| Teraspeed Modeling Services.
| http://www.teraspeed.com
[IBIS Ver]   3.2
[Comment Char] |_char
[File Name]   lpc1788fbd208.ibs
[File Rev]   3.0
[Source]  Measured and created by Teraspeed Consulting Group LLC
[Date]   04-01-2011
[Notes]   Quality Check of this IBIS model: Model Passes IBIS Check
   Model parses into ICX IS. Simulation done with Hyperlynx.
   1. MIN TYP MAX information is based on Temperature and Voltage
   characteristics only.
   2. Package data measured using Tektronix IConnect Software.
[Disclaimer]
| NXP Semiconductors warrants and represents that the IBIS models
| identified herein are owned by NXP Semiconductors (NXP).  The
| models provided are not warranted as fully representing all of the
| operating characteristics and specifications of the semiconductor
| products to which the models relate.  Moreover, unless there is a
| signed, written agreement to the contrary, these models are furnished
| on an "as is" basis without support or warranty of any kind, either
| expressed or implied, regarding the use thereof, and NXP
| specifically disclaims all implied warranties of merchantability and
| fitness of the models for any purpose.
| NXP does not assume any liability arising out of the application
| or use of these IBIS models including infringement of patents and
| copyrights, nor does NXP convey any license under its patents and
| copyrights or the rights of others.
| NXP provides IBIS models as a service to our customers.  You and
| your company shall not distribute, convey, sell, or give these models
| to anyone else without receiving prior written permission from
| NXP.
[Copyright]  NXP Semiconductors 2011. All rights reserved.
|   LPC177x_8x (208 LQFP package) IBIS Model
|   IBIS Model Created by Teraspeed Consulting Group
|   www.teraspeed.com
[Component] LPC1788FBD208
[Manufacturer] NXP Semiconductors
[Package]
| variable   typ   min   max
| lqfp208
R_pkg  1.000E-02  1.000E-02  1.000E-02
L_pkg  8.067E-09  6.742E-09  9.392E-09
C_pkg  1.248E-12  1.080E-12  1.417E-12
[Pin] signal_name  model_name  R_pin  L_pin C_pin
1   P3_12   io_pad   1.000E-02  9.392E-09  1.417E-12
2   JTAG_TDO   tri_pad   1.000E-02  9.286E-09  1.404E-12
3   P3_3   io_pad   1.000E-02  9.180E-09  1.390E-12
4   JTAG_TDI   in_pu   1.000E-02  9.074E-09  1.377E-12
5   P3_28   io_pad   1.000E-02  8.968E-09  1.363E-12
6   JTAG_TMS   in_pu   1.000E-02  8.862E-09  1.350E-12
7   P3_13   io_pad   1.000E-02  8.756E-09  1.336E-12
8   JTAG_*TRST   in_pu   1.000E-02  8.650E-09  1.323E-12
9   P5_0   io_pad   1.000E-02  8.544E-09  1.309E-12
10   JTAG_TCK   in_tck   1.000E-02  8.438E-09  1.296E-12
11   P3_29   io_pad   1.000E-02  8.332E-09  1.282E-12
12   P0_26   io_pad   1.000E-02  8.226E-09  1.269E-12
13   P3_4   io_pad   1.000E-02  8.120E-09  1.255E-12
14   P0_25   io_pad   1.000E-02  8.014E-09  1.242E-12
15   Vdd(3v3)   POWER   1.000E-02  7.908E-09  1.228E-12
16   P0_24   io_pad   1.000E-02  7.802E-09  1.215E-12
17   P3_5   io_pad   1.000E-02  7.696E-09  1.201E-12
18   P0_23   io_pad   1.000E-02  7.590E-09  1.188E-12
19   P3_30   io_pad   1.000E-02  7.484E-09  1.174E-12
20   Vdda   POWER   1.000E-02  7.378E-09  1.161E-12
21   P3_14   io_pad   1.000E-02  7.272E-09  1.147E-12
22   Vssa   GND   1.000E-02  7.166E-09  1.134E-12
23   P3_6   io_pad   1.000E-02  7.060E-09  1.120E-12
24   VREFP   term   1.000E-02  6.954E-09  1.107E-12
25   P3_31   io_pad   1.000E-02  6.848E-09  1.093E-12
26   Vdd(reg)(3v3)   POWER   1.000E-02  6.742E-09  1.080E-12
27   P3_7   io_pad   1.000E-02  6.742E-09  1.080E-12
28   P3_15   io_pad   1.000E-02  6.848E-09  1.093E-12
29   *RSTOUT   out_pad   1.000E-02  6.954E-09  1.107E-12
30   P5_1   io_pad   1.000E-02  7.060E-09  1.120E-12
31   P2_30   io_pad   1.000E-02  7.166E-09  1.134E-12
32   Vss(reg)   GND   1.000E-02  7.272E-09  1.147E-12
33   VSS   GND   1.000E-02  7.378E-09  1.161E-12
34   RTCX1   term   1.000E-02  7.484E-09  1.174E-12
35   *RESET   in_resetb   1.000E-02  7.590E-09  1.188E-12
36   RTCX2   term   1.000E-02  7.696E-09  1.201E-12
37   RTC_ALARM   rtc_alarm   1.000E-02  7.802E-09  1.215E-12
38   Vbat   POWER   1.000E-02  7.908E-09  1.228E-12
39   P2_31   io_pad   1.000E-02  8.014E-09  1.242E-12
40   P1_31   io_pad   1.000E-02  8.120E-09  1.255E-12
41   P0_12   io_pad   1.000E-02  8.226E-09  1.269E-12
42   P1_30   io_pad   1.000E-02  8.332E-09  1.282E-12
43   P2_29   io_pad   1.000E-02  8.438E-09  1.296E-12
44   XTAL1   term   1.000E-02  8.544E-09  1.309E-12
45   P0_13   io_pad   1.000E-02  8.650E-09  1.323E-12
46   XTAL2   term   1.000E-02  8.756E-09  1.336E-12
47   P2_27   io_pad   1.000E-02  8.862E-09  1.350E-12
48   P0_28   od2_pad   1.000E-02  8.968E-09  1.363E-12
49   P2_28   io_pad   1.000E-02  9.074E-09  1.377E-12
50   P0_27   od2_pad   1.000E-02  9.180E-09  1.390E-12
51   P0_31   io_pad   1.000E-02  9.286E-09  1.404E-12
52   USB_D2N   io_pad   1.000E-02  9.392E-09  1.417E-12
53   P2_24   io_pad   1.000E-02  9.392E-09  1.417E-12
54   P2_25   io_pad   1.000E-02  9.286E-09  1.404E-12
55   P3_26   io_pad   1.000E-02  9.180E-09  1.390E-12
56   P3_25   io_pad   1.000E-02  9.074E-09  1.377E-12
57   P2_26   io_pad   1.000E-02  8.968E-09  1.363E-12
58   P3_24   io_pad   1.000E-02  8.862E-09  1.350E-12
59   P2_18   io_pad   1.000E-02  8.756E-09  1.336E-12
60   Vdd(3v3)   POWER   1.000E-02  8.650E-09  1.323E-12
61   P0_29   io_pad   1.000E-02  8.544E-09  1.309E-12
62   P0_30   io_pad   1.000E-02  8.438E-09  1.296E-12
63   VSS   GND   1.000E-02  8.332E-09  1.282E-12
64   P2_23   io_pad   1.000E-02  8.226E-09  1.269E-12
65   P3_23   io_pad   1.000E-02  8.120E-09  1.255E-12
66   P1_18   io_pad   1.000E-02  8.014E-09  1.242E-12
67   P2_19   io_pad   1.000E-02  7.908E-09  1.228E-12
68   P1_19   io_pad   1.000E-02  7.802E-09  1.215E-12
69   P0_14   io_pad   1.000E-02  7.696E-09  1.201E-12
70   P1_20   io_pad   1.000E-02  7.590E-09  1.188E-12
71   Vdd(3v3)   POWER   1.000E-02  7.484E-09  1.174E-12
72   P1_21   io_pad   1.000E-02  7.378E-09  1.161E-12
73   P2_20   io_pad   1.000E-02  7.272E-09  1.147E-12
74   P1_22   io_pad   1.000E-02  7.166E-09  1.134E-12
75   P4_0   io_pad   1.000E-02  7.060E-09  1.120E-12
76   P1_23   io_pad   1.000E-02  6.954E-09  1.107E-12
77   VSS   GND   1.000E-02  6.848E-09  1.093E-12
78   P1_24   io_pad   1.000E-02  6.742E-09  1.080E-12
79   P4_1   io_pad   1.000E-02  6.742E-09  1.080E-12
80   P1_25   io_pad   1.000E-02  6.848E-09  1.093E-12
81   P2_21   io_pad   1.000E-02  6.954E-09  1.107E-12
82   P1_26   io_pad   1.000E-02  7.060E-09  1.120E-12
83   P4_2   io_pad   1.000E-02  7.166E-09  1.134E-12
84   Vss(reg)   GND   1.000E-02  7.272E-09  1.147E-12
85   P2_22   io_pad   1.000E-02  7.378E-09  1.161E-12
86   Vdd(reg)(3v3)   POWER   1.000E-02  7.484E-09  1.174E-12
87   P2_16   io_pad   1.000E-02  7.590E-09  1.188E-12
88   P1_27   io_pad   1.000E-02  7.696E-09  1.201E-12
89   Vdd(3v3)   POWER   1.000E-02  7.802E-09  1.215E-12
90   P1_28   io_pad   1.000E-02  7.908E-09  1.228E-12
91   P2_14   io_pad   1.000E-02  8.014E-09  1.242E-12
92   P1_29   io_pad   1.000E-02  8.120E-09  1.255E-12
93   VSS   GND   1.000E-02  8.226E-09  1.269E-12
94   P0_0   io_pad   1.000E-02  8.332E-09  1.282E-12
95   P2_17   io_pad   1.000E-02  8.438E-09  1.296E-12
96   P0_1   io_pad   1.000E-02  8.544E-09  1.309E-12
97   P4_3   io_pad   1.000E-02  8.650E-09  1.323E-12
98   P0_10   io_pad   1.000E-02  8.756E-09  1.336E-12
99   P2_15   io_pad   1.000E-02  8.862E-09  1.350E-12
100  P0_11   io_pad   1.000E-02  8.968E-09  1.363E-12
101  P4_16   io_pad   1.000E-02  9.074E-09  1.377E-12
102  P2_13   io_pad   1.000E-02  9.180E-09  1.390E-12
103  P4_4   io_pad   1.000E-02  9.286E-09  1.404E-12
104  P4_17   io_pad   1.000E-02  9.392E-09  1.417E-12
105  P4_18   io_pad   1.000E-02  9.392E-09  1.417E-12
106  P2_12   io_pad   1.000E-02  9.286E-09  1.404E-12
107  P4_5   io_pad   1.000E-02  9.180E-09  1.390E-12
108  P2_11   io_pad   1.000E-02  9.074E-09  1.377E-12
109  P4_20   io_pad   1.000E-02  8.968E-09  1.363E-12
110  P2_10   io_pad   1.000E-02  8.862E-09  1.350E-12
111  P4_19   io_pad   1.000E-02  8.756E-09  1.336E-12
112  Vdd(3v3)   POWER   1.000E-02  8.650E-09  1.323E-12
113  P4_6   io_pad   1.000E-02  8.544E-09  1.309E-12
114  VSS   GND   1.000E-02  8.438E-09  1.296E-12
115  P4_21   io_pad   1.000E-02  8.332E-09  1.282E-12
116  P0_22   io_pad   1.000E-02  8.226E-09  1.269E-12
117  P5_2   od1_pad   1.000E-02  8.120E-09  1.255E-12
118  P0_21   io_pad   1.000E-02  8.014E-09  1.242E-12
119  P4_26   io_pad   1.000E-02  7.908E-09  1.228E-12
120  P0_20   io_pad   1.000E-02  7.802E-09  1.215E-12
121  P4_7   io_pad   1.000E-02  7.696E-09  1.201E-12
122  P0_19   io_pad   1.000E-02  7.590E-09  1.188E-12
123  P4_22   io_pad   1.000E-02  7.484E-09  1.174E-12
124  P0_18   io_pad   1.000E-02  7.378E-09  1.161E-12
125  Vdd(3v3)   POWER   1.000E-02  7.272E-09  1.147E-12
126  P0_17   io_pad   1.000E-02  7.166E-09  1.134E-12
127  P4_8   io_pad   1.000E-02  7.060E-09  1.120E-12
128  P0_15   io_pad   1.000E-02  6.954E-09  1.107E-12
129  P4_23   io_pad   1.000E-02  6.848E-09  1.093E-12
130  P0_16   io_pad   1.000E-02  6.742E-09  1.080E-12
131  P4_9   io_pad   1.000E-02  6.742E-09  1.080E-12
132  P2_9   io_pad   1.000E-02  6.848E-09  1.093E-12
133  VSS   GND   1.000E-02  6.954E-09  1.107E-12
134  P2_8   io_pad   1.000E-02  7.060E-09  1.120E-12
135  P4_10   io_pad   1.000E-02  7.166E-09  1.134E-12
136  P2_7   io_pad   1.000E-02  7.272E-09  1.147E-12
137  P3_16   io_pad   1.000E-02  7.378E-09  1.161E-12
138  P2_6   io_pad   1.000E-02  7.484E-09  1.174E-12
139  P4_27   io_pad   1.000E-02  7.590E-09  1.188E-12
140  P2_5   io_pad   1.000E-02  7.696E-09  1.201E-12
141  P5_3   od1_pad   1.000E-02  7.802E-09  1.215E-12
142  P2_4   io_pad   1.000E-02  7.908E-09  1.228E-12
143  P3_17   io_pad   1.000E-02  8.014E-09  1.242E-12
144  P2_3   io_pad   1.000E-02  8.120E-09  1.255E-12
145  P4_11   io_pad   1.000E-02  8.226E-09  1.269E-12
146  Vdd(3v3)   POWER   1.000E-02  8.332E-09  1.282E-12
147  P1_13   io_pad   1.000E-02  8.438E-09  1.296E-12
148  VSS   GND   1.000E-02  8.544E-09  1.309E-12
149  P4_12   io_pad   1.000E-02  8.650E-09  1.323E-12
150  P2_2   io_pad   1.000E-02  8.756E-09  1.336E-12
151  P3_18   io_pad   1.000E-02  8.862E-09  1.350E-12
152  P2_1   io_pad   1.000E-02  8.968E-09  1.363E-12
153  P1_7   io_pad   1.000E-02  9.074E-09  1.377E-12
154  P2_0   io_pad   1.000E-02  9.180E-09  1.390E-12
155  P4_13   io_pad   1.000E-02  9.286E-09  1.404E-12
156  P1_5   io_pad   1.000E-02  9.392E-09  1.417E-12
157  P1_12   io_pad   1.000E-02  9.392E-09  1.417E-12
158  P0_9   io_pad   1.000E-02  9.286E-09  1.404E-12
159  P4_14   io_pad   1.000E-02  9.180E-09  1.390E-12
160  P0_8   io_pad   1.000E-02  9.074E-09  1.377E-12
161  P3_19   io_pad   1.000E-02  8.968E-09  1.363E-12
162  P0_7   io_pad   1.000E-02  8.862E-09  1.350E-12
163  P1_11   io_pad   1.000E-02  8.756E-09  1.336E-12
164  P0_6   io_pad   1.000E-02  8.650E-09  1.323E-12
165  Vdd(3v3)   POWER   1.000E-02  8.544E-09  1.309E-12
166  P0_5   io_pad   1.000E-02  8.438E-09  1.296E-12
167  P3_20   io_pad   1.000E-02  8.332E-09  1.282E-12
168  P0_4   io_pad   1.000E-02  8.226E-09  1.269E-12
169  VSS   GND   1.000E-02  8.120E-09  1.255E-12
170  P4_28   io_pad   1.000E-02  8.014E-09  1.242E-12
171  P1_6   io_pad   1.000E-02  7.908E-09  1.228E-12
172  Vss(reg)   GND   1.000E-02  7.802E-09  1.215E-12
173  P4_15   io_pad   1.000E-02  7.696E-09  1.201E-12
174  Vdd(reg)(3v3)   POWER   1.000E-02  7.590E-09  1.188E-12
175  P3_21   io_pad   1.000E-02  7.484E-09  1.174E-12
176  P4_29   io_pad   1.000E-02  7.378E-09  1.161E-12
177  P1_3   io_pad   1.000E-02  7.272E-09  1.147E-12
178  P1_17   io_pad   1.000E-02  7.166E-09  1.134E-12
179  P4_25   io_pad   1.000E-02  7.060E-09  1.120E-12
180  P1_16   io_pad   1.000E-02  6.954E-09  1.107E-12
181  Vdd(3v3)   POWER   1.000E-02  6.848E-09  1.093E-12
182  P1_15   io_pad   1.000E-02  6.742E-09  1.080E-12
183  P4_24   io_pad   1.000E-02  6.742E-09  1.080E-12
184  P1_14   io_pad   1.000E-02  6.848E-09  1.093E-12
185  P1_2   io_pad   1.000E-02  6.954E-09  1.107E-12
186  P1_10   io_pad   1.000E-02  7.060E-09  1.120E-12
187  P4_30   io_pad   1.000E-02  7.166E-09  1.134E-12
188  P1_9   io_pad   1.000E-02  7.272E-09  1.147E-12
189  VSS   GND   1.000E-02  7.378E-09  1.161E-12
190  P1_8   io_pad   1.000E-02  7.484E-09  1.174E-12
191  P3_8   io_pad   1.000E-02  7.590E-09  1.188E-12
192  P1_4   io_pad   1.000E-02  7.696E-09  1.201E-12
193  P4_31   io_pad   1.000E-02  7.802E-09  1.215E-12
194  P1_1   io_pad   1.000E-02  7.908E-09  1.228E-12
195  P3_22   io_pad   1.000E-02  8.014E-09  1.242E-12
196  P1_0   io_pad   1.000E-02  8.120E-09  1.255E-12
197  P3_0   io_pad   1.000E-02  8.226E-09  1.269E-12
198  Vdd(3v3)   POWER   1.000E-02  8.332E-09  1.282E-12
199  P3_9   io_pad   1.000E-02  8.438E-09  1.296E-12
200  VSS   GND   1.000E-02  8.544E-09  1.309E-12
201  P3_1   io_pad   1.000E-02  8.650E-09  1.323E-12
202  P0_2   io_pad   1.000E-02  8.756E-09  1.336E-12
203  P3_27   io_pad   1.000E-02  8.862E-09  1.350E-12
204  P0_3   io_pad   1.000E-02  8.968E-09  1.363E-12
205  P3_10   io_pad   1.000E-02  9.074E-09  1.377E-12
206  P5_4   io_pad   1.000E-02  9.180E-09  1.390E-12
207  P3_2   io_pad   1.000E-02  9.286E-09  1.404E-12
208  P3_11   io_pad   1.000E-02  9.392E-09  1.417E-12
[Model Selector]  in_pu
pu_2.5v   input w/int pull up,vdd=2.5v
pu_3.3v   input w/int pull up,vdd=3.3v
[Model Selector]  in_resetb
reset_2.5v   reset input w/int pull up,vdd=2.5v
reset_3.3v   reset input w/int pull up,vdd=3.3v
[Model Selector]  in_tck
tck_2.5v   tck input,vdd=2.5v
tck_3.3v   tck input,vdd=3.3v
[Model Selector]  io_pad
io_2.5v   io pin,vdd=2.5v
io_3.3v   io pin,vdd=3.3v
io_pd_2.5v  io pin w/int pull dwn,vdd=2.5v
io_pd_3.3v  io pin w/int pull dwn,vdd=3.3v
io_pu_2.5v  io pin w/int pull up,vdd=2.5v
io_pu_3.3v  io pin w/int pull up,vdd=3.3v
[Model Selector]  od1_pad
od1_2.5v   open drain1 io pin,vdd=2.5v
od1_3.3v   open drain1 io pin,vdd=3.3v
od1_pd_2.5v  open drain1 io pin w/int pull dwn,vdd=2.5v
od1_pd_3.3v  open drain1 io pin w/int pull dwn,vdd=3.3v
od1_pu_2.5v  open drain1 io pin w/int pull up,vdd=2.5v
od1_pu_3.3v  open drain1 io pin w/int pull up,vdd=3.3v
[Model Selector]  od2_pad
od2_2.5v  open drain2 io pin,vdd=2.5v
od2_3.3v  open drain2 io pin,vdd=3.3v
od2_pd_2.5v  open drain2 io pin w/int pull dwn,vdd=2.5v
od2_pd_3.3v  open drain2 io pin w/int pull dwn,vdd=3.3v
od2_pu_2.5v  open drain2 io pin w/int pull up,vdd=2.5v
od2_pu_3.3v  open drain2 io pin w/int pull up,vdd=3.3v
[Model Selector]  out_pad
out_2.5v   output pin,vdd=2.5v
out_3.3v   output pin,vdd=3.3v
[Model Selector]  tri_pad
tri_2.5v  3-state output pin,vdd=2.5v
tri_3.3v  3-state output pin,vdd=3.3v
[Model] term
Model_type Terminator
C_comp  0pF 0pF 0pF
| variable typ   min   max
[Voltage Range]   3.30000V  3.00000V  3.60000V
[POWER Clamp Reference]  3.30000V  3.00000V  3.60000V
[GND Clamp Reference]   0.00000V  0.00000V  0.00000V
[Temperature Range]   25   85   -40
| Models and submodels in the file (30): pu_2.5v (Input), pu_3.3v (Input), reset_2.5v (Input), reset_3.3v (Input), tck_2.5v (Input), tck_3.3v (Input), io_2.5v (I/O), io_pd_2.5v (I/O), io_pu_2.5v (I/O), io_3.3v (I/O), io_pd_3.3v (I/O), io_pu_3.3v (I/O), od1_2.5v (I/O_open_drain), od1_pd_2.5v (I/O_open_drain), od1_pu_2.5v (I/O_open_drain), od1_3.3v (I/O_open_drain), od1_pd_3.3v (I/O_open_drain), od1_pu_3.3v (I/O_open_drain), od2_2.5v (I/O_open_drain), od2_pd_2.5v (I/O_open_drain), od2_pu_2.5v (I/O_open_drain), od2_3.3v (I/O_open_drain), od2_pd_3.3v (I/O_open_drain), od2_pu_3.3v (I/O_open_drain), out_2.5v (Output), out_3.3v (Output), tri_2.5v (3-state), tri_3.3v (3-state), rtc_alarm (Output), term (Terminator)
